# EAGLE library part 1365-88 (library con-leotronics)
DUAL ROW STRAIGHT HEADER 1364 SERIES. 1.27mm x 1.27mm. Without Fixing Post. SMT Source: http://www.leotronics.co.uk/Conexcon/Data%20Sheets/sec.%20A/1364ing.pdf
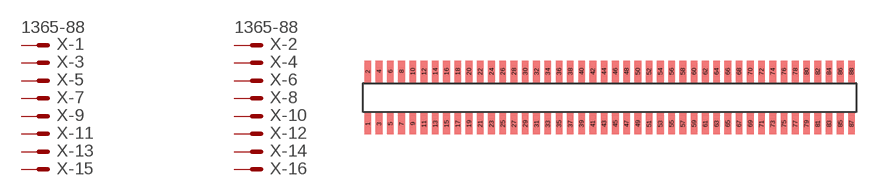
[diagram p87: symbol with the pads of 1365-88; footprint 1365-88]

Designator prefix X; gates -1=MVAL -2=MVAL -3=M -4=M -5=M -6=M -7=M -8=M -9=M -10=M -11=M -12=M -13=M -14=M -15=M -16=M -17=M -18=M -19=M -20=M -21=M -22=M -23=M -24=M -25=M -26=M -27=M -28=M -29=M -30=M -31=M -32=M -33=M -34=M -35=M -36=M -37=M -38=M -39=M -40=M -41=M -42=M -43=M -44=M -45=M -46=M -47=M -48=M -49=M -50=M -51=M -52=M -53=M -54=M -55=M -56=M -57=M -58=M -59=M -60=M -61=M -62=M -63=M -64=M -65=M -66=M -67=M -68=M -69=M -70=M -71=M -72=M -73=M -74=M -75=M -76=M -77=M -78=M -79=M -80=M -81=M -82=M -83=M -84=M -85=M -86=M -87=M -88=M

## 1365-88 (OC_FARNELL: unknown; OC_NEWARK: unknown)  [1365-88]
1  -1:S  pas
2  -2:S  pas
3  -3:S  pas
4  -4:S  pas
5  -5:S  pas
6  -6:S  pas
7  -7:S  pas
8  -8:S  pas
9  -9:S  pas
10  -10:S  pas
11  -11:S  pas
12  -12:S  pas
13  -13:S  pas
14  -14:S  pas
15  -15:S  pas
16  -16:S  pas
17  -17:S  pas
18  -18:S  pas
19  -19:S  pas
20  -20:S  pas
21  -21:S  pas
22  -22:S  pas
23  -23:S  pas
24  -24:S  pas
25  -25:S  pas
26  -26:S  pas
27  -27:S  pas
28  -28:S  pas
29  -29:S  pas
30  -30:S  pas
31  -31:S  pas
32  -32:S  pas
33  -33:S  pas
34  -34:S  pas
35  -35:S  pas
36  -36:S  pas
37  -37:S  pas
38  -38:S  pas
39  -39:S  pas
40  -40:S  pas
41  -41:S  pas
42  -42:S  pas
43  -43:S  pas
44  -44:S  pas
45  -45:S  pas
46  -46:S  pas
47  -47:S  pas
48  -48:S  pas
49  -49:S  pas
50  -50:S  pas
51  -51:S  pas
52  -52:S  pas
53  -53:S  pas
54  -54:S  pas
55  -55:S  pas
56  -56:S  pas
57  -57:S  pas
58  -58:S  pas
59  -59:S  pas
60  -60:S  pas
61  -61:S  pas
62  -62:S  pas
63  -63:S  pas
64  -64:S  pas
65  -65:S  pas
66  -66:S  pas
67  -67:S  pas
68  -68:S  pas
69  -69:S  pas
70  -70:S  pas
71  -71:S  pas
72  -72:S  pas
73  -73:S  pas
74  -74:S  pas
75  -75:S  pas
76  -76:S  pas
77  -77:S  pas
78  -78:S  pas
79  -79:S  pas
80  -80:S  pas
81  -81:S  pas
82  -82:S  pas
83  -83:S  pas
84  -84:S  pas
85  -85:S  pas
86  -86:S  pas
87  -87:S  pas
88  -88:S  pas

## Footprint 1365-88 (pad centres in mm)
DUAL ROW STRAIGHT HEADER 1364 SERIES. 1.27mm x 1.27mm. Without Fixing Post. SMT Source: http://www.leotronics.co.uk/Conexcon/Data%20Sheets/sec.%20A/1364ing.pdf
smd 0.76 x 2.4: 1 -27.305,-2.95; 2 -27.305,2.95; 3 -26.035,-2.95; 4 -26.035,2.95; 5 -24.765,-2.95; 6 -24.765,2.95; 7 -23.495,-2.95; 8 -23.495,2.95; 9 -22.225,-2.95; 10 -22.225,2.95; 11 -20.955,-2.95; 12 -20.955,2.95; 13 -19.685,-2.95; 14 -19.685,2.95; 15 -18.415,-2.95; 16 -18.415,2.95; 17 -17.145,-2.95; 18 -17.145,2.95; 19 -15.875,-2.95; 20 -15.875,2.95; 21 -14.605,-2.95; 22 -14.605,2.95; 23 -13.335,-2.95; 24 -13.335,2.95; 25 -12.065,-2.95; 26 -12.065,2.95; 27 -10.795,-2.95; 28 -10.795,2.95; 29 -9.525,-2.95; 30 -9.525,2.95; 31 -8.255,-2.95; 32 -8.255,2.95; 33 -6.985,-2.95; 34 -6.985,2.95; 35 -5.715,-2.95; 36 -5.715,2.95; 37 -4.445,-2.95; 38 -4.445,2.95; 39 -3.175,-2.95; 40 -3.175,2.95; 41 -1.905,-2.95; 42 -1.905,2.95; 43 -0.635,-2.95; 44 -0.635,2.95; 45 0.635,-2.95; 46 0.635,2.95; 47 1.905,-2.95; 48 1.905,2.95; 49 3.175,-2.95; 50 3.175,2.95; 51 4.445,-2.95; 52 4.445,2.95; 53 5.715,-2.95; 54 5.715,2.95; 55 6.985,-2.95; 56 6.985,2.95; 57 8.255,-2.95; 58 8.255,2.95; 59 9.525,-2.95; 60 9.525,2.95; 61 10.795,-2.95; 62 10.795,2.95; 63 12.065,-2.95; 64 12.065,2.95; 65 13.335,-2.95; 66 13.335,2.95; 67 14.605,-2.95; 68 14.605,2.95; 69 15.875,-2.95; 70 15.875,2.95; 71 17.145,-2.95; 72 17.145,2.95; 73 18.415,-2.95; 74 18.415,2.95; 75 19.685,-2.95; 76 19.685,2.95; 77 20.955,-2.95; 78 20.955,2.95; 79 22.225,-2.95; 80 22.225,2.95; 81 23.495,-2.95; 82 23.495,2.95; 83 24.765,-2.95; 84 24.765,2.95; 85 26.035,-2.95; 86 26.035,2.95; 87 27.305,-2.95; 88 27.305,2.95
